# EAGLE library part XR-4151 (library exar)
VOLTAGE/FREQUENCY CONVERTER
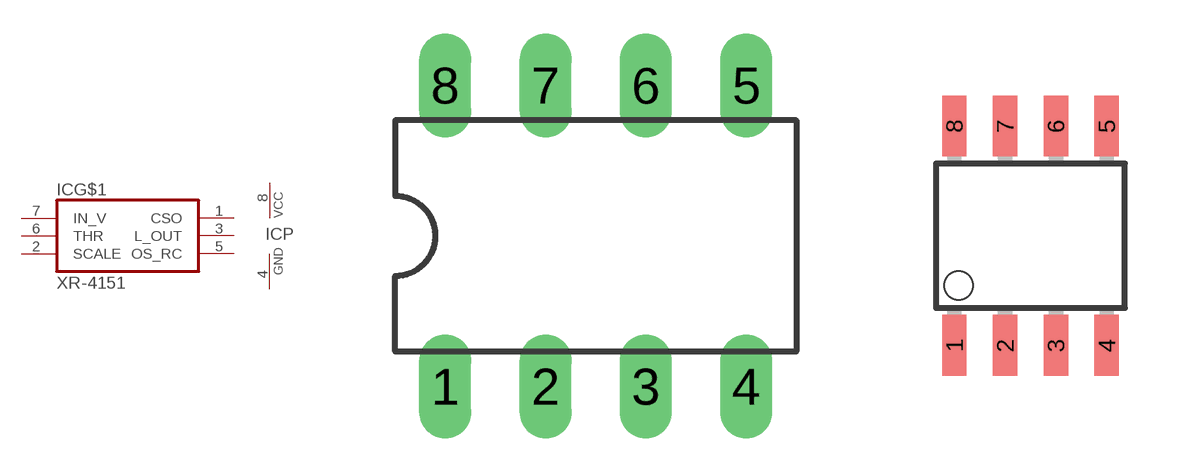
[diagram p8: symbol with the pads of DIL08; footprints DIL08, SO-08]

Designator prefix IC; gates G$1=XR-4151 P=PWRN

## XR-4151P (MPN: XR4151CP-F; OC_FARNELL: 1798672; OC_NEWARK: 24R2372)  [DIL08]
1  G$1:CSO  out
2  G$1:SCALE  pas
3  G$1:L_OUT  out
4  P:GND  pwr
5  G$1:OS_RC  pas
6  G$1:THR  in
7  G$1:IN_V  in
8  P:VCC  pwr

## XR-4151MD (OC_FARNELL: unknown; OC_NEWARK: unknown)  [SO-08]
Pads as for DIL08

## Footprint DIL08 (pad centres in mm)
Dual In Line Package
drill 0.813 long: 1 -3.81,-3.81; 2 -1.27,-3.81; 3 1.27,-3.81; 4 3.81,-3.81; 5 3.81,3.81; 6 1.27,3.81; 7 -1.27,3.81; 8 -3.81,3.81

## Footprint SO-08 (pad centres in mm)
Small Outline Package
smd 0.61 x 1.524: 1 -1.27,-2.743; 2 0,-2.743; 3 1.27,-2.743; 4 2.54,-2.743; 5 2.54,2.743; 6 1.27,2.743; 7 0,2.743; 8 -1.27,2.743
